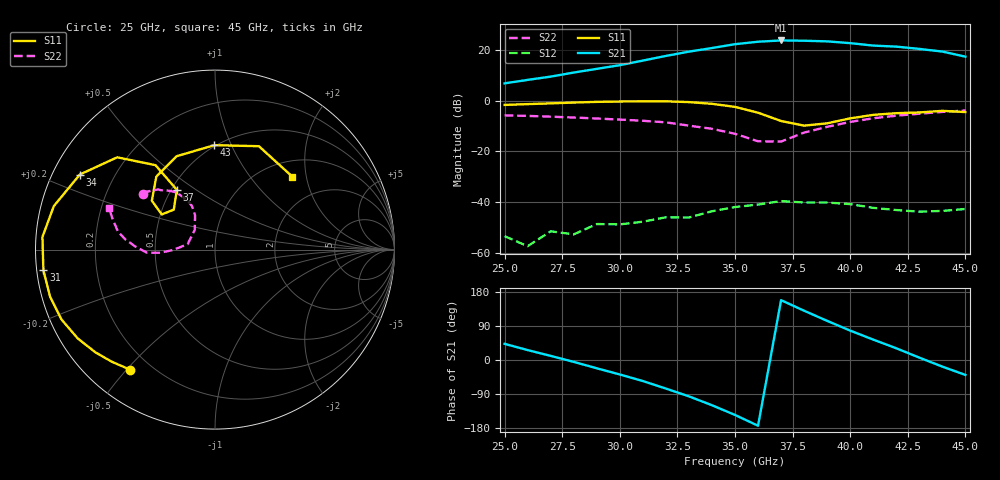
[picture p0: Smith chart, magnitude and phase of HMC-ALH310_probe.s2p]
! Hittite Microwave Corporation
! 2 Elizabeth Drive
! Chelmsford, MA 01824
! http://www.hittite.com
! Tel: 978-250-3343
! Fax: 978-250-3373
! Device:  HMC-ALH310
! Description: GaAs HEMT Low Noise Amplifier
! Frequency:  37.00 - 42.00 GHz
! Package:  DIE
! Ports:  2 RF, 4 DC
!  Pad 1 = RF In  = Port 1
!  Pad 2 = RF Out = Port 2
!  Pad 3 = Vdd
!  Pad 4 = Vgg
! Voltages:  Vdd = +2.500 Volts  Idd =  52.4 mA
!  Vgg = -0.485 Volts  Igg =  0.1 uA
! Data:  The device was measured using G-S-G Probes at the chip ports.
!  Data was collected using an calibrated network analyzer.
!  The reference plane is the pads on the amplifer chip.
! Misc:  Data collected during production testing.
!  Lot/Wafer:	 V4LM6/A-J1, 1528-029
!  Row, Column, Mod:  10, 2, 0
! Date Measured:  2007-02-26
! Date:  2011-12-06  MJV
! Note:
!  Hittite supplies this data as a sample of measured data at the package pin for
!  for this package product.  Your particular data for this product may vary.
!  Data was taken at 25 degrees C.
!  Hittite reserves the right to change this data at anytime.
# GHZ S DB R 50
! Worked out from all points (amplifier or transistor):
!   21 points, 25 GHz to 45 GHz, reference 50 ohm
!   highest |S21| = 23.7 dB at 37 GHz (marker M1)
!   |S21| within 3 dB of that: 34 GHz to 42.63 GHz (8.636 GHz wide, 22.5 % of centre)
!   unconditionally stable (mu >= 1): start of sweep to end of sweep
!   at 28 GHz: K = 8.56, MAG = 19.6 dB, |S12| = -52.7 dB
!   at 35 GHz: K = 2.12, MAG = 26.1 dB, |S12| = -42.0 dB
!   at 45 GHz: K = 3.54, MAG = 21.6 dB, |S12| = -42.7 dB
!   S11 on the Smith chart (normalised r, x): 25 GHz: 0.13, -0.51; 31 GHz: 0.02, -0.06; 34 GHz: 0.08, +0.26; 37 GHz: 0.53, +0.42; 43 GHz: 0.49, +0.86; 45 GHz: 1.33, +1.66
25  -1.73 -125.2  6.76 42.6  -53.46 139.2  -5.87 142.5
26  -1.42 -132.7  8.12 26.2  -57.39 112.3  -6.06 139.6
27  -1.12 -139.4  9.41 10.9  -51.53 164.9  -6.37 136.8
28  -0.81 -147.1  11.02 -5.0  -52.75 149.5  -6.71 133.5
29  -0.54 -155.6  12.47 -21.9  -48.67 138.3  -7.09 131.8
30  -0.40 -164.0  13.92 -38.2  -48.80 156.5  -7.51 128.7
31  -0.33 -173.1  15.73 -55.5  -47.76 155.9  -7.99 125.7
32  -0.32 175.8  17.56 -75.4  -46.00 154.4  -8.59 123.3
33  -0.63 164.9  19.26 -95.9  -46.09 161.2  -9.89 119.6
34  -1.30 150.9  20.67 -119.3  -43.64 155.2  -11.16 117.9
35  -2.51 136.7  22.19 -145.1  -41.97 142.2  -13.12 120.1
36  -4.80 125.2  23.17 -173.4  -41.00 131.8  -16.06 135.9
37  -8.07 122.5  23.66 157.9  -39.63 114.4  -16.18 168.9
38  -9.90 135.9  23.55 130.0  -40.18 99.6  -12.63 -179.5
39  -8.99 146.6  23.30 103.3  -40.20 80.5  -10.36 -176.8
40  -7.03 142.3  22.60 77.5  -40.82 66.6  -8.43 -177.3
41  -5.65 128.8  21.64 53.8  -42.29 45.1  -7.00 177.6
42  -5.00 112.4  21.23 30.9  -43.15 26.1  -5.97 173.5
43  -4.71 90.4  20.33 6.3  -43.80 -4.4  -5.20 169.5
44  -4.07 67.0  19.28 -17.5  -43.50 -8.7  -4.49 163.2
45  -4.55 43.2  17.27 -39.4  -42.74 -46.7  -3.93 158.4
